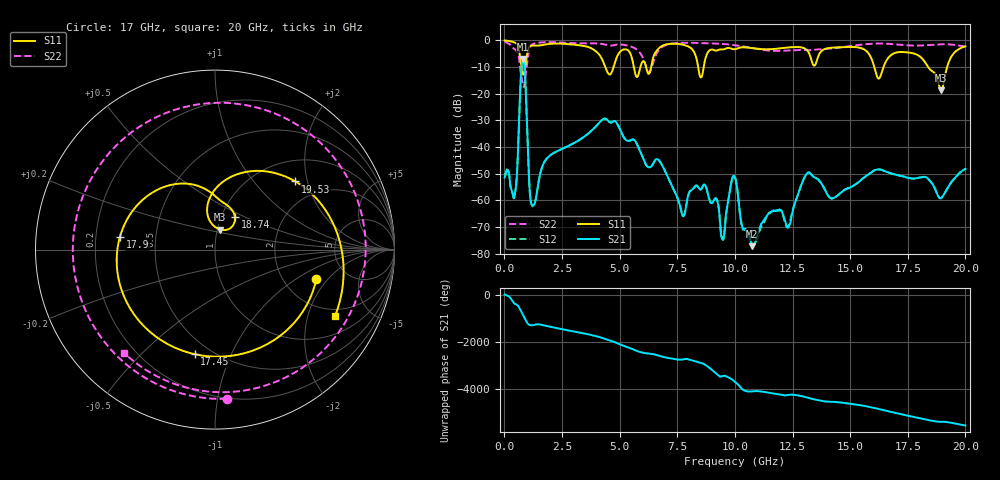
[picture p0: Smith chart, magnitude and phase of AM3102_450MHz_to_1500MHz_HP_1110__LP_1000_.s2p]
!Agilent Technologies,E8364B,MY43040894,A.07.50.67
!Agilent E8364B: A.07.50.67
!Date: Thursday, January 11, 2018 06:44:21
!Correction: S11(Full 2 Port(1,2))
!S21(Full 2 Port(1,2))
!S12(Full 2 Port(1,2))
!S22(Full 2 Port(1,2))
!S2P File: Measurements: S11, S21, S12, S22:
# Hz S  dB  R 50
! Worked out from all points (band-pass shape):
!   1601 points, 10 MHz to 20 GHz, reference 50 ohm
!   highest |S21| = -7.06 dB at 809.6 MHz (marker M1); lowest = -77.2 dB at 10.74 GHz (marker M2)
!   |S21| within 3 dB of the highest: 746 MHz to 873.4 MHz (127.4 MHz wide, 15.7 % of centre)
!   lowest |S11| = -18.7 dB at 18.95 GHz (marker M3), VSWR 1.26, Z = 51.7 + j11.7 ohm
!   |S11| at or under -10 dB: 4.375 GHz to 4.739 GHz (363.8 MHz wide, 7.98 % of centre); 16.05 GHz to 16.45 GHz (402.8 MHz wide, 2.48 % of centre); 18.38 GHz to 19.21 GHz (828.6 MHz wide, 4.41 % of centre)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
!   |S22| runs from -17.5 to -0.5 dB; largest |S21 - S12| = 0.00073
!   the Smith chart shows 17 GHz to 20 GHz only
!   S11 on the Smith chart (normalised r, x): 17 GHz: 3.01, -1.52; 17.45 GHz: 0.41, -0.74; 17.9 GHz: 0.30, +0.06; 18.74 GHz: 1.16, +0.44; 19.53 GHz: 1.46, +1.69; 20 GHz: 1.69, -3.00
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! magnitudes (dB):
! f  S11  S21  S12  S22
! 10 MHz  -0.1  -51.5  -50.7  -0.5
! 459.8 MHz  -0.9  -57.1  -57.2  -3.4
! 809.6 MHz  -12.9  -7.1  -7.1  -16.9
! 1.222 GHz  -2.0  -62.0  -62.2  -1.5
! 1.809 GHz  -1.6  -44.7  -44.6  -0.7
! 3.346 GHz  -2.0  -36.9  -36.9  -1.2
! 5.757 GHz  -13.8  -39.0  -39.0  -3.6
! 6.682 GHz  -3.2  -44.8  -44.8  -3.9
! 7.744 GHz  -1.7  -65.9  -65.8  -1.0
! 8.706 GHz  -7.4  -54.2  -54.2  -1.1
! 9.468 GHz  -3.5  -74.6  -74.6  -1.4
! 10.01 GHz  -3.4  -51.4  -51.3  -1.9
! 10.74 GHz  -3.0  -77.2  -76.2  -2.9
! 13.34 GHz  -8.0  -50.6  -50.6  -3.7
! 16.68 GHz  -6.4  -49.6  -49.6  -1.4
! 17 GHz  -4.6  -50.5  -50.5  -1.6
! 17.45 GHz  -4.5  -51.4  -51.4  -1.9
! 17.9 GHz  -5.4  -51.7  -51.6  -2.0
! 18.74 GHz  -13.5  -56.8  -56.7  -1.6
! 18.95 GHz  -18.7  -59.1  -59.2  -1.5
! 19.53 GHz  -4.6  -51.8  -51.8  -1.8
! 20 GHz  -2.3  -48.3  -48.2  -2.3
